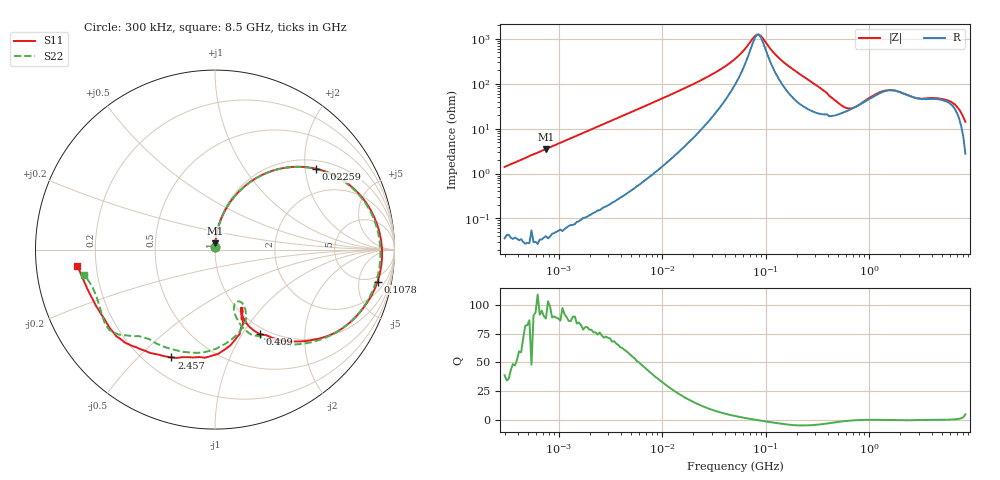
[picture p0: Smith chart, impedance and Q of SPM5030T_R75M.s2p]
! S-Parameter Data Generated by TDK Corporation
! Copyright(C) 2023 TDK Corporation.
! All Rights Reserved.
! TDK P/N: SPM5030T-R75M (Inductor)
! Property: L=750nH at 100kHz
! Size(LxWxT): 5.2x5x3mm
! Model Type: s2p (Touchstone File Format Version 1.0)
! Frequency: DC=Yes Start=0.3MHz Stop=8500MHz 225points Log-sweep
! Model Generated on Sep. 29, 2023
! Port Assignments:
!  1 ---@@@--- 2
! Applicable Conditions:
!  Temperature = 25 degC
!  DC Bias Current = 0 A
!  Small Signal Operation
! Terms and conditions regarding TDK Simulation Models
! (1)This simulation model is being provided solely for informational purposes. Please refer to the specifications of the products in terms of detailed characteristics of such products.
! (2)In no event shall TDK Corporation of any of its subsidiaries be liable for any loss or damage arising, directly or indirectly,
!  From any information contained in this simulation model, including, but not limited to loss or damages arising from any inaccuracies, omissions or errors in connection with such information.
! (3)Any and all copyrights on this simulation model are owned by TDK Corporation.
!  Duplication or redistribution of this simulation model without prior written permission from TDK Corporation is prohibited.
! (4)This simulation model is subject to any modification or change without any prior notice.
! (5)Neither TDK Corporation nor any of its subsidiaries shall make any warranty, express or implied,
!  Including but not limited to the correctness, implied warranties of merchantability and fitness for a particular purpose with respect to this simulation models.
! (6)The use of this simulation model shall be deemed to have consented to the terms and conditions hereof.
# Hz S MA R 50
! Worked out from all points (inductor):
!   224 points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, 300 kHz to 8.5 GHz, reference 50 ohm
!   read as one part in series: L = 744 nH near 314.1 kHz
!   highest Q = 94.8 at 752.4 kHz (marker M1), where L = 745 nH
!   self-resonance near 84.34 MHz
!   S11 on the Smith chart (normalised r, x): 300 kHz: 1.00, +0.03; 22.59 MHz: 1.22, +2.29; 107.8 MHz: 3.63, -8.76; 409 MHz: 0.91, -1.20; 2.457 GHz: 0.30, -0.63; 8.5 GHz: 0.13, -0.06
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300000  0.01462 89.5  0.9999 -0.9  0.998 -0.7  0.0147 90.3
752368.3  0.03517 87.5  0.9993 -2.1  0.9983 -1.9  0.03527 87.6
1721110  0.07943 84.6  0.9961 -4.7  0.9953 -4.6  0.07942 84.6
4732045  0.2127 76.4  0.9732 -12.6  0.973 -12.4  0.2127 76.4
9430415  0.3979 64.4  0.9052 -24.0  0.9054 -23.8  0.3982 64.3
2.258783e7  0.7208 38.7  0.6405 -47.2  0.6405 -47.0  0.7211 38.5
5.167171e7  0.906 11.3  0.2425 -62.7  0.2426 -62.5  0.9018 10.7
8.182903e7  0.9314 -2.6  0.07425 -14.0  0.07426 -13.8  0.9222 -3.6
8.970948e7  0.9309 -5.4  0.07914 15.8  0.0792 15.9  0.9209 -6.5
1.078202e8  0.9231 -11.1  0.1387 45.3  0.1388 45.4  0.9125 -12.5
1.630757e8  0.8704 -25.3  0.3273 49.3  0.3274 49.4  0.8601 -27.2
2.831228e8  0.6987 -47.1  0.5834 29.7  0.5836 29.8  0.6904 -50.0
4.089767e8  0.5333 -62.1  0.7181 10.4  0.7182 10.5  0.5196 -66.6
5.642308e8  0.4073 -67.5  0.7488 -7.2  0.7489 -7.0  0.3803 -72.8
7.784218e8  0.3559 -65.8  0.7058 -24.9  0.706 -24.8  0.3144 -67.5
1.232735e9  0.4227 -68.6  0.5351 -45.2  0.5353 -45.1  0.4238 -65.8
1.551304e9  0.5394 -80.7  0.4629 -52.2  0.463 -52.0  0.5082 -79.4
2.456696e9  0.648 -112.0  0.3906 -65.4  0.391 -65.3  0.6045 -113.3
3.890506e9  0.708 -130.7  0.2981 -94.5  0.2981 -94.3  0.6685 -133.9
5.884306e9  0.73 -145.1  0.22 -112.4  0.2199 -112.3  0.7379 -145.4
7.072242e9  0.7336 -155.1  0.2068 -125.0  0.2066 -124.7  0.7148 -155.0
8.5e9  0.7717 -173.1  0.1678 -141.9  0.1683 -142.0  0.7432 -169.0
